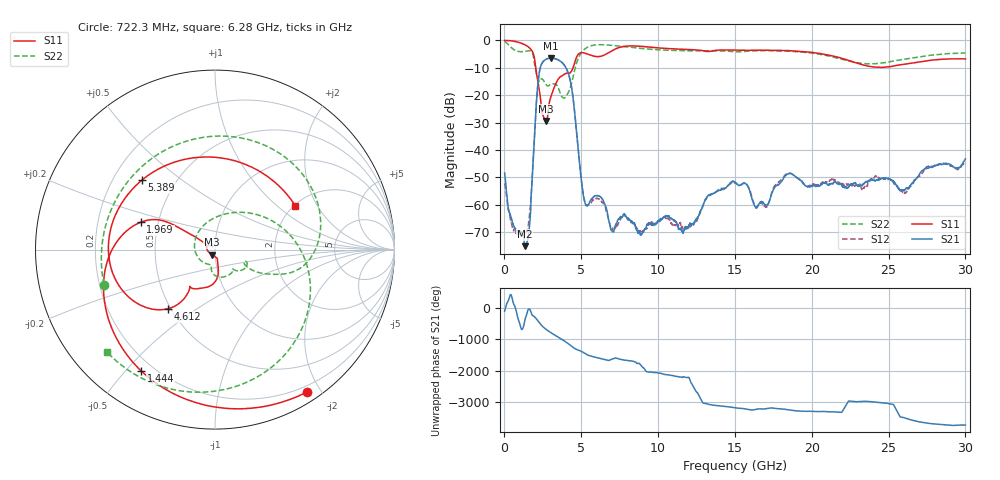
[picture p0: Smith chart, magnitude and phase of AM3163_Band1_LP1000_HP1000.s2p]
!Agilent Technologies,E8364B,MY43040894,A.07.50.67
!Agilent E8364B: A.07.50.67
!Date: Thursday, August 20, 2020 11:21:48
!Correction: S11(Full 2 Port(1,2))
!S21(Full 2 Port(1,2))
!S12(Full 2 Port(1,2))
!S22(Full 2 Port(1,2))
!S2P File: Measurements: S11, S21, S12, S22:
# Hz S  dB  R 50
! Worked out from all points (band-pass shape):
!   3201 points, 10 MHz to 30 GHz, reference 50 ohm
!   highest |S21| = -6.53 dB at 3.037 GHz (marker M1); lowest = -75.1 dB at 1.322 GHz (marker M2)
!   |S21| within 3 dB of the highest: 2.356 GHz to 3.949 GHz (1.592 GHz wide, 50.5 % of centre)
!   lowest |S11| = -29.4 dB at 2.7 GHz (marker M3), VSWR 1.07, Z = 48.1 - j2.73 ohm
!   |S11| at or under -10 dB: 2.034 GHz to 4.47 GHz (2.436 GHz wide, 74.9 % of centre)
!   |S22| runs from -21.1 to -0.5 dB; largest |S21 - S12| = 0.0055
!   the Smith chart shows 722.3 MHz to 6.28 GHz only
!   S11 on the Smith chart (normalised r, x): 722.3 MHz: 0.13, -1.83; 1.444 GHz: 0.15, -0.55; 1.969 GHz: 0.40, +0.15; 4.612 GHz: 0.48, -0.39; 5.389 GHz: 0.32, +0.37; 6.28 GHz: 2.02, +1.34
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1e7  -0.10 -5.1  -48.38 -113.6  -52.19 127.3  -0.48 -19.7
7.222625e8  -0.50 -57.0  -68.77 -24.4  -69.73 62.4  -3.76 -162.4
1.322062e9  -1.65 -109.1  -75.07 -55.1  -70.36 -80.9  -4.08 104.4
1.443897e9  -2.03 -121.2  -74.09 155.5  -69.52 -178.5  -3.95 84.9
1.968722e9  -7.12 159.7  -32.92 65.0  -33.06 64.6  -9.06 -23.0
2.268622e9  -18.19 147.3  -11.77 -116.3  -11.77 -116.4  -15.01 -24.5
2.699728e9  -29.43 -123.0  -6.97 35.4  -6.97 35.4  -16.13 -46.5
3.037116e9  -20.36 -79.6  -6.53 -78.9  -6.54 -78.9  -15.98 -54.3
3.636916e9  -13.34 -102.6  -7.64 103.2  -7.64 103.3  -19.46 -101.5
4.611591e9  -7.47 -128.7  -28.63 133.4  -28.62 133.3  -9.95 36.2
5.014581e9  -4.52 179.6  -51.38 51.3  -51.61 51.3  -4.46 -28.0
5.389456e9  -5.01 136.2  -60.31 -56.9  -60.27 -54.4  -2.60 -69.4
6.279784e9  -5.85 28.8  -57.20 -179.4  -58.51 -177.2  -1.63 -136.5
7.441897e9  -2.71 -104.5  -65.17 170.9  -66.46 169.8  -2.12 163.4
8.454059e9  -2.09 179.6  -67.15 85.2  -66.59 66.6  -2.74 120.6
1.000979e10  -2.80 99.6  -65.78 85.7  -65.81 75.5  -3.50 61.4
1.220281e10  -3.45 11.4  -67.12 95.4  -67.40 -71.2  -3.87 -14.0
1.5005e10  -3.57 -71.6  -51.69 56.0  -52.02 58.6  -4.23 -93.1
2.000958e10  -4.44 163.2  -53.07 -53.7  -52.51 -50.2  -4.70 136.8
2.276491e10  -8.06 60.0  -52.08 -104.2  -52.91 -101.2  -8.01 21.0
2.500479e10  -9.71 -62.4  -50.40 -169.0  -50.64 -169.2  -7.97 -92.2
3e10  -6.85 110.6  -43.20 -129.3  -45.05 -134.7  -4.66 103.1
